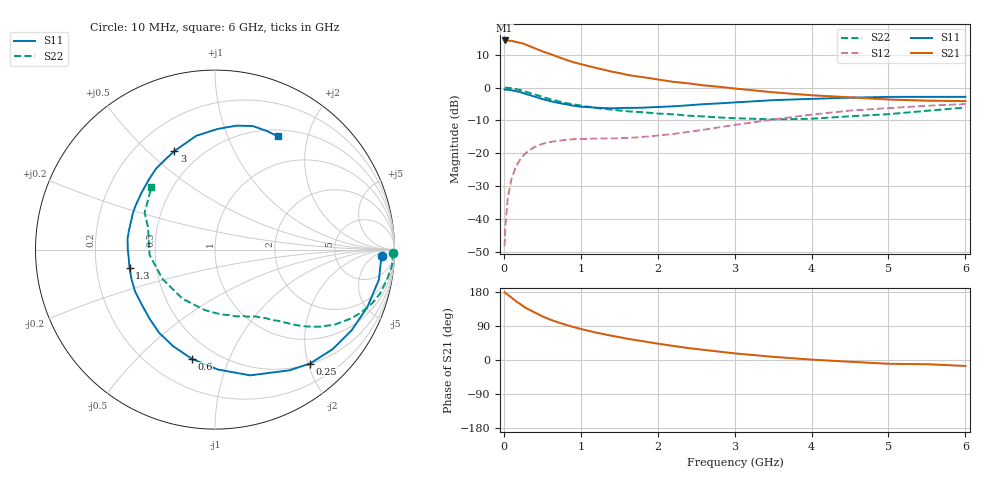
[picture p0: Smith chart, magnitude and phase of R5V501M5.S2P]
! SIEMENS Small Signal Semiconductors
! BFR183
! Si NPN RF Bipolar Junction Transistor in SOT23
! VCE = 0.5 V  IC = 1.5 mA
! Common Emitter S-Parameters:  May  1996
# GHz  S  MA  R  50
!  f  S11  S21  S12  S22
! GHz  MAG  ANG  MAG  ANG  MAG  ANG  MAG  ANG
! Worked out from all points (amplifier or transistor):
!   36 points, 10 MHz to 6 GHz, reference 50 ohm
!   highest |S21| = 14.3 dB at 10 MHz (marker M1)
!   |S21| within 3 dB of that: start of sweep to 468.4 MHz
!   unconditionally stable (mu >= 1): 1.411 GHz to 3.67 GHz; 5.853 GHz to end of sweep
!   at 250 MHz: K = 0.20, MSG = 17.1 dB, |S12| = -20.7 dB
!   at 1.4 GHz: K = 1.00, MSG = 10.1 dB, |S12| = -15.4 dB
!   at 6 GHz: K = 1.00, MAG = 0.2 dB, |S12| = -5.0 dB
!   S11 on the Smith chart (normalised r, x): 10 MHz: 22, -11; 250 MHz: 0.51, -2.03; 600 MHz: 0.37, -0.74; 1.3 GHz: 0.35, -0.09; 3 GHz: 0.36, +0.61; 6 GHz: 0.58, +1.54
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0.01  0.9313 -2.1  5.18 178.8  0.0039 89.2  0.9938 -1.0
0.02  0.9265 -4.3  5.15 176.7  0.0078 85.1  0.9907 -2.0
0.05  0.9284 -10.4  5.122 172.2  0.0205 84.1  0.9906 -5.1
0.1  0.9074 -20.6  5.116 164.7  0.0413 77.8  0.9732 -9.9
0.15  0.8841 -30.6  4.936 156.4  0.0597 71.8  0.9519 -14.9
0.25  0.8267 -50.2  4.658 142.2  0.0918 61.6  0.8876 -23.1
0.3  0.7898 -58.4  4.415 135.9  0.1047 57.3  0.8527 -26.6
0.4  0.7277 -74.3  3.949 125.6  0.1249 49.7  0.7868 -32.1
0.5  0.6685 -88.6  3.544 115.3  0.139 43.8  0.7228 -36.5
0.6  0.622 -102.0  3.234 106.9  0.1485 39.0  0.6666 -40.0
0.7  0.5866 -113.4  2.927 99.7  0.1549 35.7  0.622 -42.7
0.8  0.5585 -123.9  2.652 93.3  0.1595 33.0  0.5838 -44.9
0.9  0.5302 -133.4  2.429 87.4  0.1641 31.0  0.5567 -46.6
1.1  0.5028 -152.3  2.116 77.0  0.1668 28.8  0.5106 -50.3
1.3  0.487 -167.8  1.86 68.2  0.1684 28.2  0.4737 -53.6
1.6  0.4911 172.8  1.56 56.3  0.172 30.1  0.4364 -58.7
2.2  0.5176 142.3  1.221 37.2  0.1968 36.5  0.3919 -71.9
3  0.5935 112.5  0.966 17.5  0.2702 39.7  0.3417 -99.6
3.5  0.6425 99.4  0.846 8.4  0.3271 36.5  0.3281 -123.4
4.5  0.7008 80.2  0.709 -4.6  0.446 24.2  0.366 -175.4
5.5  0.7211 66.5  0.631 -11.1  0.5283 10.8  0.4431 152.2
6  0.722 61.1  0.622 -15.7  0.5599 2.2  0.4964 135.5
